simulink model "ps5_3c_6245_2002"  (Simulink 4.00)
settings: Solver=ode45  StartTime=0.0  StopTime=30.0  RelTol=1e-3
libraries: cstblocks x6, simulink3 x1

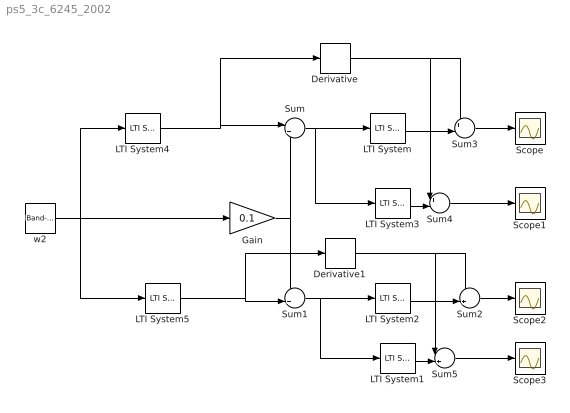
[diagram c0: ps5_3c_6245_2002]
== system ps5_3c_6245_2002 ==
  Derivative : Derivative
  Derivative1 : Derivative
  Gain : Gain  Gain=0.1  Multiplication=Element-wise(K.*u)  SaturateOnIntegerOverflow=on
  LTI System : cstblocks/LTI System  sys=H1  IC=0
  LTI System1 : cstblocks/LTI System  sys=H1  IC=0
  LTI System2 : cstblocks/LTI System  sys=H10  IC=0
  LTI System3 : cstblocks/LTI System  sys=H10  IC=0
  LTI System4 : cstblocks/LTI System  sys=W1  IC=0
  LTI System5 : cstblocks/LTI System  sys=W10  IC=0
  Scope{,1..3} (4 alike) : Scope
  Sum : Sum  Inputs=|++  SaturateOnIntegerOverflow=on
  Sum1 : Sum  Inputs=++|  SaturateOnIntegerOverflow=on
  Sum2 : Sum  Inputs=-+|  SaturateOnIntegerOverflow=on
  Sum3 : Sum  Inputs=+-|  SaturateOnIntegerOverflow=on
  Sum4 : Sum  Inputs=+-|  SaturateOnIntegerOverflow=on
  Sum5 : Sum  Inputs=-+|  SaturateOnIntegerOverflow=on
  w2 : simulink3/Sources/Band-Limited White Noise  Cov=[0.1]  Ts=0.001  seed=[23341]
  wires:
  LTI System4/1 -> Sum/1, Derivative/1
  Gain/1 -> Sum/2, Sum1/1
  LTI System5/1 -> Sum1/2, Derivative1/1
  Sum/1 -> LTI System/1, LTI System3/1
  Sum1/1 -> LTI System2/1, LTI System1/1
  LTI System/1 -> Sum3/2
  LTI System3/1 -> Sum4/2
  LTI System2/1 -> Sum2/2
  LTI System1/1 -> Sum5/2
  Sum3/1 -> Scope/1
  Sum4/1 -> Scope1/1
  Sum2/1 -> Scope2/1
  Sum5/1 -> Scope3/1
  w2/1 -> LTI System4/1, Gain/1, LTI System5/1
  Derivative/1 -> Sum3/1, Sum4/1
  Derivative1/1 -> Sum2/1, Sum5/1
